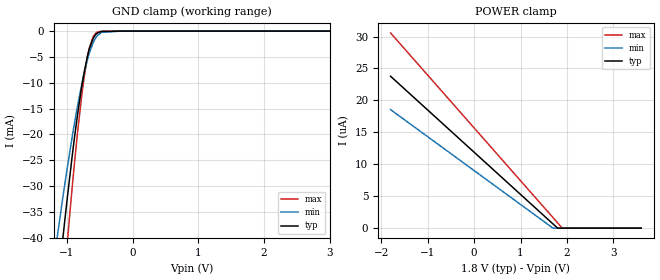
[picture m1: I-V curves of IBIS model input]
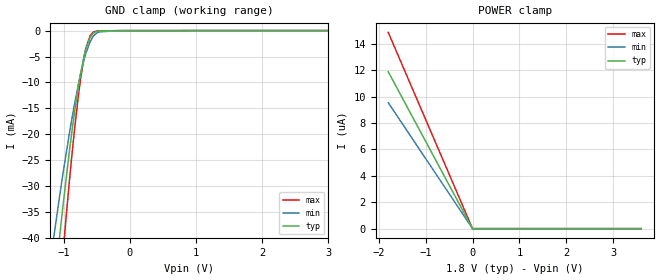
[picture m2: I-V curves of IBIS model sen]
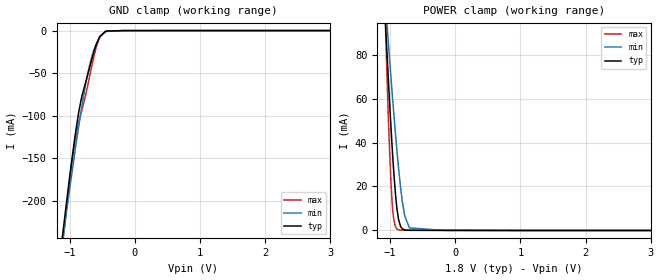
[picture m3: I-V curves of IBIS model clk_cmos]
|Texas Instruments Incorporated
| Quad-Channel Integrated Analog Front End for Automotive Radar Applications
| Marketing part#   Digital Voltage Range   Package-type   #pins
| AFE5401   1.7V-3.6V   QFN   64
[IBIS Ver]   4.1
[File name]   afe5401.ibs
[File Rev]   1.0
[Date]   2/18/2014
[Source]
| Texas Instruments Incorporated.
| Analog-eLab Design Center, HPA
| 12500 TI Blvd
| Dallas, TX -75243
[Notes]   Revision History:
| Rev 1.0: 2/18/2014
| - Initial version of the model
| - Model generated from simulations in TISPICE
| - Model matched to SPICE simulation
| - C_comp although listed in numerical order of value are
|   obtained from varying PVT conditions. For PVT conditions for
|   each specific value refer the buffer description under
|   respective [Model]. IBIS model user is responsible for using
|   appropriate C_comp to simulate for Signal Integrity.
|*EXCEPTION:   *
|* - For input model,There will be small leakage currents in POWER clamp   *
|* - IV-table because of the resistor (RES3T_NPL_SIBLK) connected to the pad  *
|* - For sen model,There will be small leakage currents in GROUND clamp   *
|* - IV-table because of the resistor (RES3T_NPL_SIBLK) connected to the pad  *
|* - For clk_cmos and clkin_diff* models,There will be small leakage   *
|* - currents in POWER and GROUND clamp IV-table because of the resistor   *
|* - (RES3T_NPL_SIBLK) connected between CLKP and CLKM.   *
[Disclaimer]
| This model is designed as an aid for customers of Texas Instruments.
| TI and its licensors and suppliers make no warranties, either expressed
| or implied, with respect to this  model, including the warranties of
| merchantability or fitness for a particular purpose. The model is
| provided solely on an "as is" basis. The entire risk as to its quality
| and performance is with the customer.
[Copyright]
(C) Copyright 2014 Texas Instruments Incorporated.All rights reserved.
|   AFE5401RGC
[Component]   AFE5401RGC
[Manufacturer]   TI
[Package]   |64 QFN  -  RGC package
|   typ   min   max
R_pkg   0.16638   0.08903   0.21557
L_pkg   2.19973nH   1.76900nH   2.84471nH
C_pkg   0.23530pF   0.19862pF   0.30827pF
[Pin]  signal_name   model_name   R_pin   L_pin   C_pin
1   IN1P_AUX   NC   0.21235   2.80578nH  0.28156pF
2   IN1M_AUX   NC   0.18459   2.40086nH  0.26768pF
3   IN1P   NC   0.17098   2.21481nH  0.24755pF
4   IN1M   NC   0.15198   1.95802nH  0.22705pF
5   IN2P_AUX   NC   0.14019   1.79926nH  0.21465pF
6   IN2M_AUX   NC   0.12822   1.63864nH  0.19732pF
7   IN2P   NC   0.12266   1.56423nH  0.19124pF
8   IN2M   NC   0.12346   1.57493nH  0.19523pF
9   IN3P_AUX   NC   0.12822   1.63853nH  0.20024pF
10   IN3M_AUX   NC   0.14019   1.79913nH  0.20924pF
11   IN3P   NC   0.15516   2.00084nH  0.22499pF
12   IN3M   NC   0.17465   2.26426nH  0.23633pF
13   IN4P_AUX   NC   0.15447   1.99153nH  0.22268pF
14   IN4M_AUX   NC   0.17385   2.25384nH  0.24703pF
15   IN4P   NC   0.19354   2.52221nH  0.27583pF
16   IN4M   NC   0.22178   2.93508nH  0.28725pF
17   VCM   NC   0.20430   2.69535nH  0.25028pF
18   AVDD3   POWER   0.09499   1.90426nH  0.31612pF
19   AVDD18   POWER   0.06288   1.78742nH  0.35075pF
20   AVSS   GND   0.09183   1.82315nH  0.31403pF
21   CLKINP   CLK   0.09000   1.79451nH  0.30827pF
22   CLKINM   CLK   0.08903   1.76900nH  0.30745pF
23   AVSS   GND   0.08912   1.72560nH  0.31796pF
24   AVDD18   POWER   0.06053   1.69354nH  0.33200pF
25   TRIG   input   0.17639   2.28431nH  0.22954pF
26   DSYNC1   DSYNC   0.17927   2.32243nH  0.23946pF
27   DSYNC2   DSYNC   0.18673   2.42272nH  0.24450pF
28   DVDD18   POWER   0.19586   2.54605nH  0.24934pF
29   DVSS   GND   0.20602   2.68350nH  0.26034pF
30   DVDD18   POWER   0.10851   2.23689nH  0.31972pF
31   DRVSS   GND   0.19344   2.51516nH  0.24487pF
32   DRVDD   POWER   0.21374   2.81793nH  0.25674pF
33   DRVDD   POWER   0.21592   2.84937nH  0.26274pF
34   DCLK   DCLK   0.19149   2.48774nH  0.25891pF
35   D[0]   DCLK   0.17472   2.25814nH  0.23624pF
36   D[1]   DCLK   0.16415   2.11443nH  0.22177pF
37   D[2]   DCLK   0.15522   1.99335nH  0.21288pF
38   D[3]   DCLK   0.14799   1.89541nH  0.20610pF
39   D[4]   DCLK   0.14272   1.82433nH  0.20114pF
40   D[5]   DCLK   0.13980   1.78471nH  0.19862pF
41   D[6]   DCLK   0.13922   1.77693nH  0.20041pF
42   D[7]   DCLK   0.14276   1.82473nH  0.20374pF
43   D[8]   DCLK   0.14813   1.89734nH  0.20956pF
44   D[9]   DCLK   0.15947   2.05106nH  0.22033pF
45   D[10]   DCLK   0.16938   2.18533nH  0.23067pF
46   D[11]   DCLK   0.18557   2.40545nH  0.24658pF
47   D_GPO[1]   D_GPO   0.19800   2.57627nH  0.25583pF
48   D_GPO[0]   D_GPO   0.21557   2.84471nH  0.25547pF
49   DRVSS   GND   0.22216   2.93380nH  0.26849pF
50   DRVDD   POWER   0.10252   2.06005nH  0.33128pF
51   DVDD18   POWER   0.10305   2.09094nH  0.33748pF
52   DVSS   GND   0.06681   1.92296nH  0.36530pF
53   SDOUT   SDOUT   0.19621   2.55125nH  0.24610pF
54   SEN   sen   0.18960   2.46205nH  0.24079pF
55   SDATA   input   0.18523   2.40333nH  0.23677pF
56   SCLK   input   0.18327   2.37743nH  0.23495pF
57   RESET   input   0.18381   2.38543nH  0.23541pF
58   NC   NC   0.18682   2.42703nH  0.23780pF
59   STBY   input   0.19219   2.50054nH  0.23626pF
60   NC   NC   0.18569   2.41146nH  0.23441pF
61   AVSS   GND   0.06381   1.80505nH  0.36062pF
62   AVDD18   POWER   0.06494   1.82063nH  0.38721pF
63   AVSS   GND   0.09930   1.99680nH  0.34126pF
64   VCM   NC   0.21459   2.83802nH  0.26074pF
[Diff_pin]   inv_pin   vdiff   tdelay_typ   tdelay_min   tdelay_max
21   22   0.2V   0   0   0
|   Model Selectors
[Model Selector] CLK
clkin_diff_p   1.8V differential input
clkin_diff_n   1.8V differential input
clk_cmos   1.8V digital input CMOS mode
[Model Selector] SDOUT
sdout_3p3   3.3V digital output
sdout_1p8   1.8V digital output
[Model Selector] D_GPO
d_gpo_3p3   3.3V digital tristate with FAST_DGPO set to 0
d_gpo_1p8   1.8V digital tristate with FAST_DGPO set to 0
d_gpo_f_3p3  3.3V digital tristate with FAST_DGPO set to 1
d_gpo_f_1p8  1.8V digital tristate with FAST_DGPO set to 1
[Model Selector] DCLK
dclk_3p3   3.3V digital tristate
dclk_1p8   1.8V digital tristate
[Model Selector] DSYNC
dsync_3p3   3.3V digital output
dsync_1p8   1.8V digital output
| Models and submodels in the file (15): input (Input), sen (Input), clk_cmos (Input), clkin_diff_p (Input), clkin_diff_n (Input), sdout_1p8 (Output), sdout_3p3 (Output), d_gpo_1p8 (3-state), d_gpo_3p3 (3-state), d_gpo_f_1p8 (3-state), d_gpo_f_3p3 (3-state), dclk_1p8 (3-state), dclk_3p3 (3-state), dsync_1p8 (Output), dsync_3p3 (Output)
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|   input Model
[Model]   input
Model_type   Input
Vinl = 0.54
Vinh = 1.26
|   typ   min   max
|   (nom PVT)   (fast PVT)   (slow PVT)
C_comp   1.275e-12   1.236e-12   1.316e-12
[Model spec]
|subparameter
Vinl   0.54   0.51   0.57
Vinh   1.26   1.19   1.33
| Where nom  PVT is Nominal Process, 1.8V, 27C
|   Fast PVT is Strong Process,  1.9V, -40C
|   Slow PVT is Weak Process,   1.7V, 125C
[Voltage Range]   1.8   1.7   1.9
|Junction Temperature
[Temperature Range]   27   125   -40
[Power Clamp Reference]   1.8   1.7   1.9
[GND Clamp Reference]   0   0   0
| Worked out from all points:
|   GND clamp passes 1 mA (typ) near -0.58 V on its own axis
[GND Clamp]
|   Voltage   I(typ)   I(min)   I(max)
-1.8V     -193.6mA   -124.3mA   -262.8mA
-1.152V   -51.15mA   -40.23mA   -65.29mA
-1.062V   -40.1mA    -32.17mA   -51.03mA
-1.006V   -33.52mA   -27.35mA   -42.46mA
-916mV    -23.73mA   -20.14mA   -29.62mA
-882mV    -20.3mA    -17.59mA   -25.09mA
-740.9mV  -8.187mA   -8.287mA   -9.168mA
-660mV    -3.458mA   -4.286mA   -3.266mA
-559.3mV  -616.5uA   -1.246mA   -373.8uA
-470.6mV  -73.81uA   -264uA     -28.25uA
-180mV    -1.194uA   -1.193uA   -1.487uA
3.6V      0A         0A         0A
[POWER Clamp]
|   Voltage   I(typ)   I(min)   I(max)
-1.8V     23.79uA    18.56uA    30.57uA
1.699V    670nA      0A         1.664uA
1.798V    11.89nA    0A         841.1nA
1.899V    0A         0A         0A
3.6V      0A         0A         0A
|   sen Model
[Model]   sen
Model_type   Input
Vinl = 0.54
Vinh = 1.26
|   typ   min   max
|   (nom PVT)   (fast PVT)   (slow PVT)
C_comp   1.275e-12   1.236e-12   1.316e-12
[Model spec]
|subparameter
Vinl   0.54   0.51   0.57
Vinh   1.26   1.19   1.33
| Where nom  PVT is Nominal Process, 1.8V, 27C
|   Fast PVT is Strong Process,  1.9V, -40C
|   Slow PVT is Weak Process,   1.7V, 125C
[Voltage Range]   1.8   1.7   1.9
|Junction Temperature
[Temperature Range]   27   125   -40
[Power Clamp Reference]   1.8   1.7   1.9
[GND Clamp Reference]   0   0   0
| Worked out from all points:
|   GND clamp passes 1 mA (typ) near -0.58 V on its own axis
[GND Clamp]
|   Voltage   I(typ)   I(min)   I(max)
-1.8V     -193.6mA   -124.3mA   -262.8mA
-1.152V   -51.15mA   -40.23mA   -65.29mA
-1.062V   -40.1mA    -32.17mA   -51.03mA
-1.006V   -33.52mA   -27.36mA   -42.46mA
-916mV    -23.74mA   -20.15mA   -29.62mA
-882mV    -20.3mA    -17.59mA   -25.09mA
-740.9mV  -8.194mA   -8.292mA   -9.177mA
-660mV    -3.465mA   -4.291mA   -3.277mA
-559.3mV  -626.5uA   -1.253mA   -387.9uA
-470.6mV  -85.36uA   -272.3uA   -43.78uA
-180mV    -13.09uA   -10.21uA   -17.19uA
3.6V      0A         0A         0A
[POWER Clamp]
|   Voltage   I(typ)   I(min)   I(max)
-1.8V     11.89uA    9.549uA    14.87uA
-1.4mV    0A         0A         11.58nA
-700uV    0A         0A         0A
3.6V      0A         0A         0A
|   clk_cmos Model
[Model]   clk_cmos
Model_type   Input
Vinl = 0.45
Vinh = 1.35
|   typ   min   max
|   (nom PVT)   (fast PVT)   (slow PVT)
C_comp   3.036e-12   2.656e-12   3.427e-12
[Model spec]
|subparameter
Vinl   0.45   0.425   0.475
Vinh   1.35   1.275   1.425
| Where nom  PVT is Nominal Process, 1.8V, 27C
|   Fast PVT is Strong Process,  1.9V, -40C
|   Slow PVT is Weak Process,   1.7V, 125C
[Voltage Range]   1.8   1.7   1.9
|Junction Temperature
[Temperature Range]   27   125   -40
[Power Clamp Reference]   1.8   1.7   1.9
[GND Clamp Reference]   0   0   0
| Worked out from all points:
|   GND clamp passes 1 mA (typ) near -0.45 V on its own axis
|   POWER clamp passes 1 mA (typ) near -0.82 V on its own axis
[GND Clamp]
|   Voltage   I(typ)   I(min)   I(max)
-1.8V     -724.2mA   -669.6mA   -781.3mA
-1.125V   -252.7mA   -258.5mA   -264.5mA
-1.029V   -190.7mA   -203.3mA   -197.2mA
-967.8mV  -153.9mA   -169.7mA   -158.4mA
-920.3mV  -126.8mA   -144.2mA   -132.6mA
-870.1mV  -101.1mA   -118.1mA   -112.2mA
-820.8mV  -80.81mA   -93.77mA   -96.6mA
-749.3mV  -59.96mA   -61.71mA   -74.82mA
-647.4mV  -30.71mA   -27.74mA   -37.92mA
-544.1mV  -8.303mA   -8.713mA   -9.331mA
-449.1mV  -1.057mA   -1.649mA   -926.5uA
3.6V      0A         0A         0A
[POWER Clamp]
|   Voltage   I(typ)   I(min)   I(max)
-1.8V     579.6mA    427.8mA    962.6mA
-1.074V   95.57mA    104.3mA    94.98mA
-1.042V   76.57mA    91.02mA    63.76mA
-1.008V   57.47mA    77.36mA    35.2mA
-986.8mV  46.44mA    69.18mA    21.27mA
-948.6mV  28.23mA    54.71mA    5.82mA
-895.6mV  9.795mA    36.1mA     628uA
-873mV    5.251mA    28.89mA    277.5uA
-813.6mV  768.3uA    13.19mA    102.3uA
-774.9mV  242.1uA    6.439mA    91.81uA
-703.5mV  78.41uA    1.182mA    86.96uA
3.6V      0A         0A         0A
